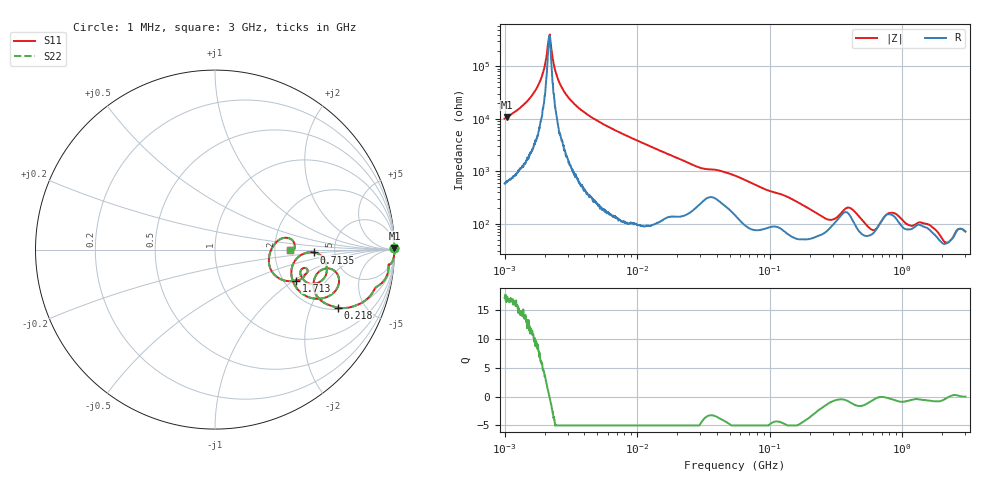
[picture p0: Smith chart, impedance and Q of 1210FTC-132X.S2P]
!s-Parameter Generated by FASTRON Sdn. Bhd.
!FASTRON P/N : 1210FTC-132X
!Keysight Technologies: E4991B_MY54100416_A.01.15
!Date created: Mon Dec 11 10:00:43 2023
!Version  : Rev00 Mon Dec 11 10:00:43 2023
!Data & Calibration Information:
!Freq	S11	S21	S12	S22
!PortZ  Port1:50+j0  Port2:50+j0
!When reading reference impedance value at option line is always used.
! Remarks : This data is being provided solely for informational purposes.
# Hz S dB R 50
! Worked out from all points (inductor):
!   1601 points, 1 MHz to 3 GHz, reference 50 ohm
!   read as one part in series: L = 1.26 mH near 1.041 MHz
!   highest Q = 17.1 at 1.046 MHz (marker M1), where L = 1.64 mH
!   self-resonance near 2.172 MHz
!   S11 on the Smith chart (normalised r, x): 1 MHz: open; 218 MHz: 2.10, -3.17; 713.5 MHz: 3.45, -0.16; 1.713 GHz: 2.32, -1.04; 3 GHz: 2.42, +0.00
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1000000  -0.01 0.6  -40.07 -86.1  -40.07 -86.1  -0.01 0.6
1046065  -0.00 0.5  -40.69 -86.2  -40.69 -86.2  -0.00 0.5
1725357  -0.00 0.2  -51.27 -83.6  -51.27 -83.6  -0.00 0.2
1935809  -0.00 0.1  -57.27 -78.1  -57.27 -78.1  -0.00 0.1
2182827  -0.00 -0.0  -71.87 6.3  -71.87 6.3  -0.00 -0.0
2424692  -0.00 -0.1  -57.96 79.4  -57.96 79.4  -0.00 -0.1
2626804  -0.00 -0.1  -53.20 83.7  -53.20 83.7  -0.00 -0.1
3804036  -0.00 -0.4  -43.28 87.6  -43.28 87.6  -0.00 -0.4
1.447069e7  -0.02 -2.2  -28.16 85.4  -28.16 85.4  -0.02 -2.2
5.477226e7  -0.24 -6.6  -18.59 73.2  -18.59 73.2  -0.24 -6.6
2.083556e8  -2.14 -24.6  -7.22 48.4  -7.22 48.4  -2.14 -24.6
2.179536e8  -2.42 -25.3  -6.91 45.6  -6.91 45.6  -2.42 -25.3
2.827291e8  -4.57 -21.4  -6.04 25.6  -6.04 25.6  -4.57 -21.4
3.453811e8  -4.06 -9.7  -8.04 15.4  -8.04 15.4  -4.06 -9.7
4.135554e8  -2.91 -16.1  -8.64 32.4  -8.64 32.4  -2.91 -16.1
5.077325e8  -4.44 -26.7  -5.40 30.1  -5.40 30.1  -4.44 -26.7
6.049187e8  -7.06 -16.5  -4.60 12.4  -4.60 12.4  -7.06 -16.5
7.135306e8  -5.18 -1.6  -6.94 2.0  -6.94 2.0  -5.18 -1.6
7.925923e8  -4.16 -6.3  -8.17 10.1  -8.17 10.1  -4.16 -6.3
1.712864e9  -6.33 -20.9  -4.80 17.4  -4.80 17.4  -6.33 -20.9
2.167021e9  -10.33 -8.9  -3.09 3.8  -3.09 3.8  -10.33 -8.9
3e9  -7.63 0.0  -4.66 -0.0  -4.66 -0.0  -7.63 0.0
